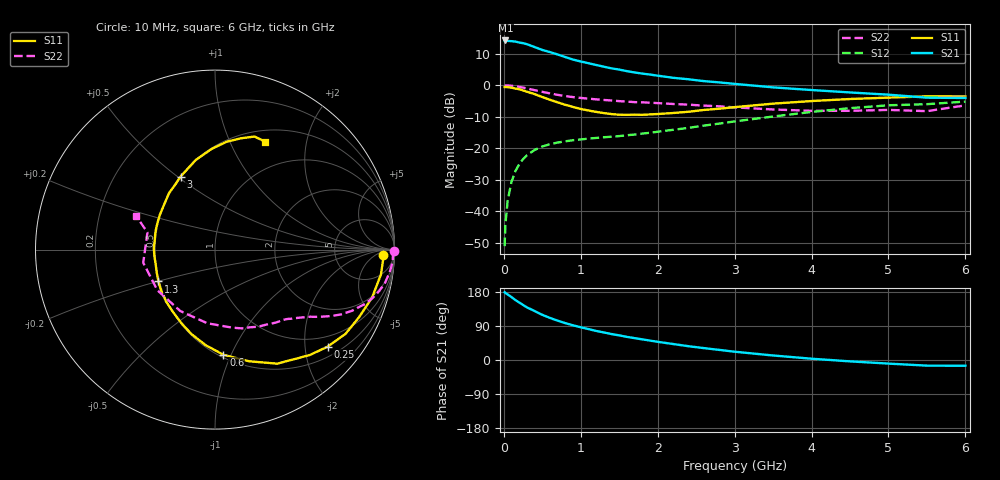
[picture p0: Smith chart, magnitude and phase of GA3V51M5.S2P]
! Infineon Technologies  Discrete & RF Semiconductors
! BF775
! Si NPN RF Bipolar Junction Transistor in SOT23
! VCE = 3.5 V  IC = 1.5 mA
! Common Emitter S-Parameters:  May  1996
# GHz  S  MA  R  50
!  f  S11  S21  S12  S22
! GHz  MAG  ANG  MAG  ANG  MAG  ANG  MAG  ANG
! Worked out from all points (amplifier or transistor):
!   36 points, 10 MHz to 6 GHz, reference 50 ohm
!   highest |S21| = 14.2 dB at 20 MHz (marker M1)
!   |S21| within 3 dB of that: start of sweep to 498.5 MHz
!   unconditionally stable (mu >= 1): 1.298 GHz to 3.847 GHz; 5.237 GHz to end of sweep
!   at 250 MHz: K = 0.24, MSG = 18.4 dB, |S12| = -23.4 dB
!   at 1.4 GHz: K = 1.06, MAG = 9.4 dB, |S12| = -16.3 dB
!   at 6 GHz: K = 1.00, MAG = 0.2 dB, |S12| = -5.2 dB
!   S11 on the Smith chart (normalised r, x): 10 MHz: 25, -12; 250 MHz: 0.73, -2.51; 600 MHz: 0.52, -0.94; 1.3 GHz: 0.49, -0.20; 3 GHz: 0.50, +0.51; 6 GHz: 0.63, +1.36
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0.01  0.9368 -1.7  5.069 178.9  0.0028 87.9  0.9985 -0.6
0.02  0.9382 -3.5  5.137 177.0  0.0061 90.3  0.992 -1.5
0.05  0.935 -8.5  5.053 172.9  0.0149 85.5  0.9927 -3.8
0.1  0.9152 -16.9  5.004 166.0  0.0295 79.8  0.9812 -7.4
0.15  0.8867 -25.1  4.93 158.1  0.0435 75.1  0.9651 -11.1
0.25  0.8282 -40.8  4.652 145.2  0.0674 66.2  0.9183 -17.1
0.3  0.7896 -48.1  4.484 138.9  0.0776 62.8  0.8901 -19.8
0.4  0.7238 -61.4  4.039 129.2  0.0941 56.3  0.8356 -24.1
0.5  0.6501 -73.1  3.631 119.2  0.1068 51.1  0.7867 -27.4
0.6  0.588 -85.4  3.358 111.0  0.1161 47.3  0.7429 -29.9
0.7  0.5349 -95.6  3.073 103.7  0.1234 44.6  0.7048 -32.0
0.8  0.4893 -105.4  2.796 97.3  0.1291 42.6  0.6735 -33.8
0.9  0.4531 -113.9  2.556 91.5  0.1344 41.4  0.6486 -35.2
1.1  0.3979 -133.1  2.238 81.6  0.1425 39.9  0.6128 -38.1
1.3  0.362 -150.6  1.969 72.7  0.1497 39.4  0.5846 -40.8
1.6  0.3397 -174.2  1.674 61.0  0.1611 40.9  0.5502 -45.1
2.2  0.3628 148.3  1.313 42.2  0.1964 44.3  0.5047 -56.1
3  0.4496 115.3  1.052 21.9  0.267 44.1  0.4459 -77.4
3.5  0.5107 102.1  0.926 11.9  0.3195 40.7  0.4128 -95.9
4.5  0.6052 83.7  0.769 -3.6  0.4332 29.1  0.393 -144.9
5.5  0.6674 70.7  0.635 -14.9  0.5012 12.6  0.3883 165.8
6  0.6634 65.2  0.628 -15.2  0.5511 8.0  0.4795 156.7
